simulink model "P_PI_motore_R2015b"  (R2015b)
settings: Solver=ode45  StartTime=0.0  StopTime=0.5  RelTol=1e-3
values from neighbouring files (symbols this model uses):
  A = [0,1,0,0    [labcontaut4.m]
  B = [0;1/Jm;0;0]    [labcontaut4.m]
  Kpp = 35.34    [labcontaut4.m]
  Kpv = Kiv*Tiv    [labcontaut4.m]
  Tiv = 10/wz    [labcontaut4.m]
libraries: simulink x2

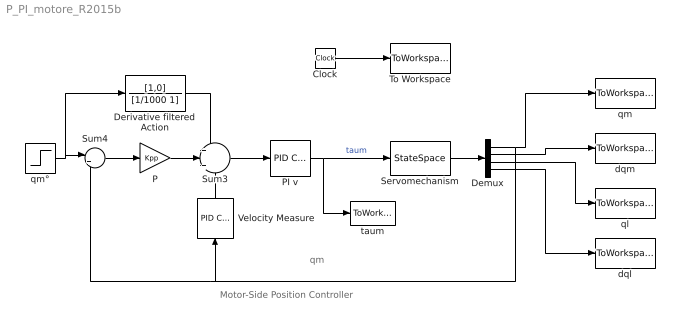
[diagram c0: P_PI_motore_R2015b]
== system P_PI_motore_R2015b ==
  note: qm
  note: Motor-Side Position Controller
  Clock : Clock
  Demux : Demux
  Derivative filtered Action : TransferFcn  Numerator=[1,0]  Denominator=[1/1000 1]
  P : Gain  Gain=Kpp
  PI v : simulink/Continuous/PID Controller  Controller=PI  TimeDomain=Continuous-time  SampleTime=-1  IntegratorMethod=Forward Euler  FilterMethod=Forward Euler  Form=Ideal  UseFilter=on  ControllerParametersSource=internal  P=Kpv  I=1/Tiv  D=0  N=100  InitialConditionSource=internal  InitialConditionForIntegrator=0  InitialConditionForFilter=0  ExternalReset=none  LimitOutput=off  UpperSaturationLimit=inf  LowerSaturationLimit=-inf  LinearizeAsGain=on  AntiWindupMode=none  Kb=1  TrackingMode=off  Kt=1  PParamMin=[]  PParamMax=[]  IParamMin=[]  IParamMax=[]  DParamMin=[]  DParamMax=[]  NParamMin=[]  NParamMax=[]  KbParamMin=[]  KbParamMax=[]  KtParamMin=[]  KtParamMax=[]  POutMin=[]  POutMax=[]  IOutMin=[]  IOutMax=[]  DOutMin=[]  DOutMax=[]  NOutMin=[]  NOutMax=[]  KbOutMin=[]  KbOutMax=[]  KtOutMin=[]  KtOutMax=[]  IntegratorOutMin=[]  IntegratorOutMax=[]  FilterOutMin=[]  FilterOutMax=[]  SumOutMin=[]  SumOutMax=[]  SumI1OutMin=[]  SumI1OutMax=[]  SumI2OutMin=[]  SumI2OutMax=[]  SumI3OutMin=[]  SumI3OutMax=[]  SumDOutMin=[]  SumDOutMax=[]  SaturationOutMin=[]  SaturationOutMax=[]  IntegratorContinuousStateAttributes=''  IntegratorStateMustResolveToSignalObject=off  IntegratorRTWStateStorageClass=Auto  FilterContinuousStateAttributes=''  FilterStateMustResolveToSignalObject=off  FilterRTWStateStorageClass=Auto  DifferentiatorICPrevScaledInput=0  DifferentiatorOutMin=[]  DifferentiatorOutMax=[]
  Servomechanism : StateSpace  A=A  B=B  C=eye(4)  D=zeros(4,1)  X0=[0;0;0;0]
  Sum3 : Sum  Inputs=+|+|-
  Sum4 : Sum  Inputs=|+-
  To Workspace : ToWorkspace  VariableName=t  SampleTime=-1
  Velocity Measure : simulink/Continuous/PID Controller  Controller=PD  TimeDomain=Continuous-time  SampleTime=-1  IntegratorMethod=Forward Euler  FilterMethod=Forward Euler  Form=Parallel  UseFilter=on  ControllerParametersSource=internal  P=0  I=1  D=1  N=1000  InitialConditionSource=internal  InitialConditionForIntegrator=0  InitialConditionForFilter=0  ExternalReset=none  LimitOutput=off  UpperSaturationLimit=inf  LowerSaturationLimit=-inf  LinearizeAsGain=on  AntiWindupMode=none  Kb=1  TrackingMode=off  Kt=1  PParamMin=[]  PParamMax=[]  IParamMin=[]  IParamMax=[]  DParamMin=[]  DParamMax=[]  NParamMin=[]  NParamMax=[]  KbParamMin=[]  KbParamMax=[]  KtParamMin=[]  KtParamMax=[]  POutMin=[]  POutMax=[]  IOutMin=[]  IOutMax=[]  DOutMin=[]  DOutMax=[]  NOutMin=[]  NOutMax=[]  KbOutMin=[]  KbOutMax=[]  KtOutMin=[]  KtOutMax=[]  IntegratorOutMin=[]  IntegratorOutMax=[]  FilterOutMin=[]  FilterOutMax=[]  SumOutMin=[]  SumOutMax=[]  SumI1OutMin=[]  SumI1OutMax=[]  SumI2OutMin=[]  SumI2OutMax=[]  SumI3OutMin=[]  SumI3OutMax=[]  SumDOutMin=[]  SumDOutMax=[]  SaturationOutMin=[]  SaturationOutMax=[]  IntegratorContinuousStateAttributes=''  IntegratorStateMustResolveToSignalObject=off  IntegratorRTWStateStorageClass=Auto  FilterContinuousStateAttributes=''  FilterStateMustResolveToSignalObject=off  FilterRTWStateStorageClass=Auto  DifferentiatorICPrevScaledInput=0  DifferentiatorOutMin=[]  DifferentiatorOutMax=[]
  dql : ToWorkspace  VariableName=dql  SampleTime=-1
  dqm : ToWorkspace  VariableName=dqm  SampleTime=-1
  ql : ToWorkspace  VariableName=ql  SampleTime=-1
  qm : ToWorkspace  VariableName=qm  SampleTime=-1
  qm° : Step  Time=0  SampleTime=0
  taum : ToWorkspace  VariableName=taum  SampleTime=-1
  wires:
  Sum4/1 -> P/1
  qm°/1 -> Derivative filtered Action/1, Sum4/1
  P/1 -> Sum3/2
  Servomechanism/1 -> Demux/1
  Demux/3 -> ql/1
  Demux/4 -> dql/1
  Demux/1 -> qm/1, Velocity Measure/1, Sum4/2
  Demux/2 -> dqm/1
  Clock/1 -> To Workspace/1
  Sum3/1 -> PI v/1
  PI v/1 -> taum/1, Servomechanism/1  "taum"
  Velocity Measure/1 -> Sum3/3
  Derivative filtered Action/1 -> Sum3/1
